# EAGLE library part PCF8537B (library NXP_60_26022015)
Industrial LCD driver for multiplex rates up to 1:8. SPI version. The PCF8537 is a fully featured Liquid Crystal Display (LCD) driver, specifically designed for high-contrast Vertical Alignment (VA) LCD with multiplex rates up to 1:8. It generates the drive signals for any static or multiplexed LCD containing up to eight backplanes, 46 segments, and up to 352 elements. The PCF8537 features an internal charge pump with internal capacitors for on-chip generation of the LCD driving voltage. To ensure an optimal and stable contrast over the full temperature range, the PCF8537 offers a programmable temperature compensation of the LCD supply voltage. The PCF8537 can be easily connected to a microcontroller by either the two-line I2C-bus (PCF8537AH) or a three-line bidirectional SPI-bus (PCF8537BH). AAL Eindhoven MK
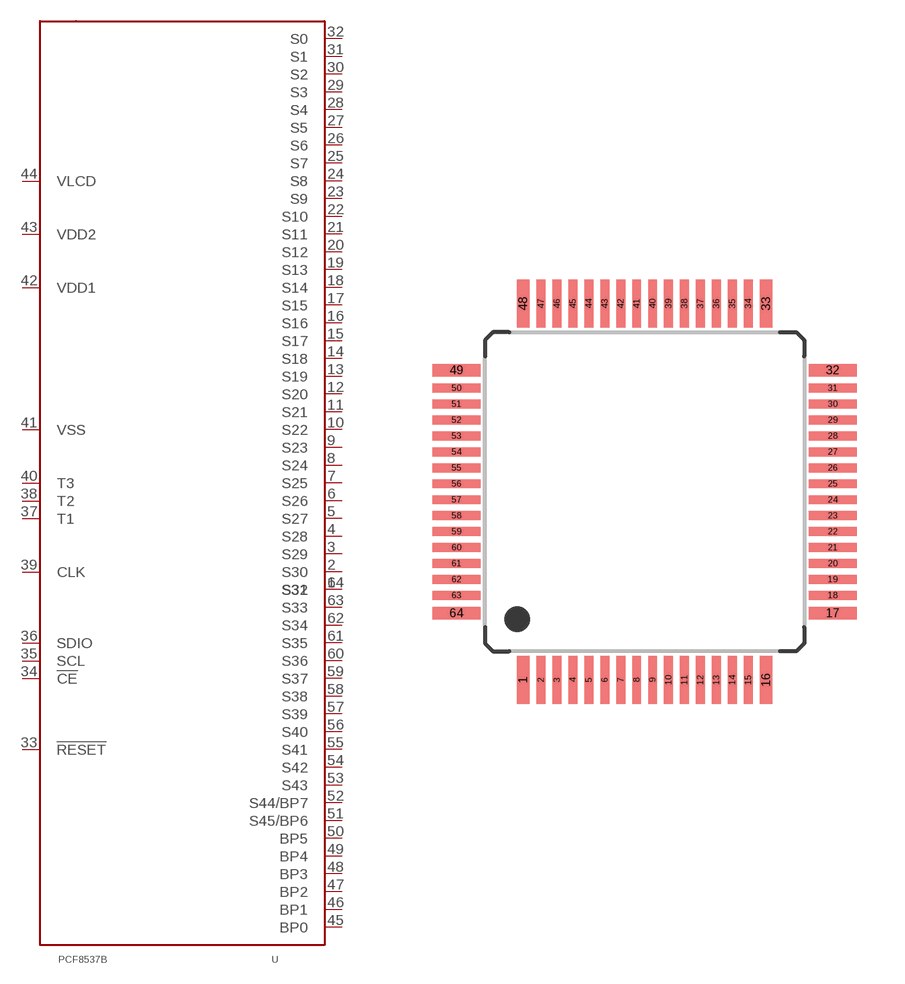
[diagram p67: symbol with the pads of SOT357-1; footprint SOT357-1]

Designator prefix U

## PCF8537B  [SOT357-1]
1  S31  out
2  S30  out
3  S29  out
4  S28  out
5  S27  out
6  S26  out
7  S25  out
8  S24  out
9  S23  out
10  S22  out
11  S21  out
12  S20  out
13  S19  out
14  S18  out
15  S17  out
16  S16  out
17  S15  out
18  S14  out
19  S13  out
20  S12  out
21  S11  out
22  S10  out
23  S9  out
24  S8  out
25  S7  out
26  S6  out
27  S5  out
28  S4  out
29  S3  out
30  S2  out
31  S1  out
32  S0  out
33  !RESET!  out
34  !CE!  out
35  SCL  out
36  SDIO  out
37  T1  out
38  T2  out
39  CLK  out
40  T3  out
41  VSS  out
42  VDD1  out
43  VDD2  out
44  VLCD  out
45  BP0  out
46  BP1  out
47  BP2  out
48  BP3  out
49  BP4  out
50  BP5  out
51  S45/BP6  out
52  S44/BP7  out
53  S43  out
54  S42  out
55  S41  out
56  S40  out
57  S39  out
58  S38  out
59  S37  out
60  S36  out
61  S35  out
62  S34  out
63  S33  out
64  S32  out

## Footprint SOT357-1 (pad centres in mm)
SOT357-1 TQFP64: plastic thin quad flat package; 64 leads; body 10 x 10 x 1.0 mm JEDEC: MS-026 IEC: 137E10 JEITA: --
smd 0.4 x 1.5: 1 -3.81,-5.9; 16 3.81,-5.9; 33 3.81,5.9; 48 -3.81,5.9
smd 0.28 x 1.5: 2 -3.25,-5.9; 3 -2.75,-5.9; 4 -2.25,-5.9; 5 -1.75,-5.9; 6 -1.25,-5.9; 7 -0.75,-5.9; 8 -0.25,-5.9; 9 0.25,-5.9; 10 0.75,-5.9; 11 1.25,-5.9; 12 1.75,-5.9; 13 2.25,-5.9; 14 2.75,-5.9; 15 3.25,-5.9; 34 3.25,5.9; 35 2.75,5.9; 36 2.25,5.9; 37 1.75,5.9; 38 1.25,5.9; 39 0.75,5.9; 40 0.25,5.9; 41 -0.25,5.9; 42 -0.75,5.9; 43 -1.25,5.9; 44 -1.75,5.9; 45 -2.25,5.9; 46 -2.75,5.9; 47 -3.25,5.9
smd 1.5 x 0.4: 17 5.9,-3.81; 32 5.9,3.81; 49 -5.9,3.81; 64 -5.9,-3.81
smd 1.5 x 0.28: 18 5.9,-3.25; 19 5.9,-2.75; 20 5.9,-2.25; 21 5.9,-1.75; 22 5.9,-1.25; 23 5.9,-0.75; 24 5.9,-0.25; 25 5.9,0.25; 26 5.9,0.75; 27 5.9,1.25; 28 5.9,1.75; 29 5.9,2.25; 30 5.9,2.75; 31 5.9,3.25; 50 -5.9,3.25; 51 -5.9,2.75; 52 -5.9,2.25; 53 -5.9,1.75; 54 -5.9,1.25; 55 -5.9,0.75; 56 -5.9,0.25; 57 -5.9,-0.25; 58 -5.9,-0.75; 59 -5.9,-1.25; 60 -5.9,-1.75; 61 -5.9,-2.25; 62 -5.9,-2.75; 63 -5.9,-3.25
